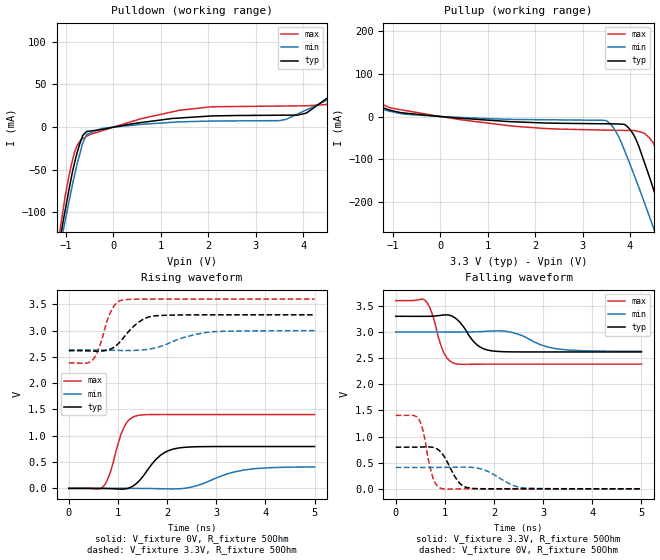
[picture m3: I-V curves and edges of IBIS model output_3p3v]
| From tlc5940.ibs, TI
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|   output_3p3v Model
[Model]   output_3p3v
Model_type   Output
Polarity   Non-Inverting
Vmeas = 1.65
Vref = 1.65
Cref = 15pF
Rref = 50
|   typ   min   max
|   (nom PVT)   (Fast PVT)   (slow PVT)
|Average
C_comp   1.731e-12   1.729e-12   1.773e-12
|ON state : BUFFER OUTPUT TURNED HIGH
|C_comp   1.838e-12   1.835e-12   1.905e-12
|OFF state: BUFFER is in LOW state
|C_comp   1.628e-12   1.621e-12   1.641e-12
| Where nom  PVT is Nominal Process, 3.3V, 65C
|   Fast PVT is Strong Process,  3.6V, -40C
|   Slow PVT is Weak Process,   3V, 125C
[Voltage Range]   3.3   3   3.6
|Ambient Temperature   25   85   -40
|Junction Temperature
[Temperature Range]   65   125   -40
[Pullup Reference]   3.3   3   3.6
[Pulldown Reference]   0   0   0
[Power Clamp Reference]   3.3   3   3.6
[GND Clamp Reference]   0   0   0
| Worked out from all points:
|   slope of the pulldown table from 0 to 0.495 V, typ, clamps not added: 104 ohm
|   slope of the pullup table from 0 to 0.495 V, typ, clamps not added: 107 ohm
|   falling waveform, V_fixture 3.3V, R_fixture 50Ohm: 20-80 % time 327ps typ, 545ps min, 229ps max; typ from 3.3 V to 2.62 V
|   rising waveform, V_fixture 0V, R_fixture 50Ohm: 20-80 % time 430ps typ, 735ps min, 270ps max; typ from 0 V to 0.796 V
|   rising waveform, V_fixture 3.3V, R_fixture 50Ohm: 20-80 % time 417ps typ, 697ps min, 255ps max; typ from 2.62 V to 3.3 V
|   falling waveform, V_fixture 0V, R_fixture 50Ohm: 20-80 % time 284ps typ, 463ps min, 183ps max; typ from 0.796 V to 0 V
[Pulldown]
|   Voltage   I(typ)   I(min)   I(max)
-3.3V     -940.2mA   -857.4mA   -1.084A
-1.139V   -135.7mA   -144.9mA   -125.6mA
-1.092V   -120.7mA   -131mA     -108.3mA
-1.046V   -105.9mA   -117.8mA   -91.31mA
-823.2mV  -42.75mA   -57.22mA   -30.01mA
-564mV    -5.078mA   -8.618mA   -10.77mA
1.398V    10.71mA    6.227mA    19.78mA
3.498V    13.98mA    7.63mA     24.69mA
4.066V    16.44mA    20.12mA    25.02mA
4.49V     33.36mA    31.46mA    26.46mA
4.814V    46.59mA    40.99mA    50.25mA
6.6V      125.7mA    93.65mA    209.8mA
[Pullup]
|   Voltage   I(typ)   I(min)   I(max)
-3.3V     110.7mA    76.62mA    210.2mA
-1.061V   14.71mA    12.28mA    20.6mA
1.538V    -12.39mA   -6.887mA   -22.73mA
3.498V    -17.16mA   -9.56mA    -32.01mA
3.759V    -17.69mA   -47mA      -32.48mA
4.019V    -33.45mA   -117.8mA   -32.94mA
4.188V    -70.87mA   -167.3mA   -35.65mA
4.487V    -168.3mA   -259.4mA   -61.5mA
4.752V    -259.4mA   -344mA     -158mA
4.926V    -322.2mA   -400.7mA   -230.3mA
5.115V    -390.5mA   -463.1mA   -311.7mA
6.6V      -960mA     -972.2mA   -980.3mA
[Ramp]
R_load = 50
|   typ   min   max
dV/dt_r   0.477664/4.29009e-10   0.244378/7.25716e-10   0.842488/2.69271e-10
dV/dt_f   0.409109/3.26691e-10   0.221026/5.38551e-10   0.728975/2.28779e-10
[Falling Waveform]
V_fixture = 3.3V
V_fixture_min = 3V
V_fixture_max = 3.6V
R_fixture = 50Ohm
|   Time   V(typ)   V(min)   V(max)
0s        3.3V       3V         3.6V
610ps     3.3V       3V         3.592V
740ps     3.303V     3V         3.354V
980ps     3.326V     3V         2.603V
1.22ns    3.26V      2.999V     2.393V
1.65ns    2.757V     3.005V     2.384V
1.94ns    2.641V     3.018V     2.385V
2.44ns    2.619V     2.973V     2.385V
3.29ns    2.618V     2.676V     2.385V
5ns       2.618V     2.632V     2.385V
[Rising Waveform]
V_fixture = 0V
V_fixture_min = 0V
V_fixture_max = 0V
R_fixture = 50Ohm
|   Time   V(typ)   V(min)   V(max)
0s        217pV      1.746nV    184.6pV
700ps     -1.346mV   318uV      34.54mV
840ps     -4.411mV   391.2uV    296.3mV
1.11ns    -13.2mV    214.7uV    1.137V
1.35ns    73.79mV    -716.1uV   1.372V
1.85ns    617.5mV    -6.212mV   1.404V
2.14ns    750.6mV    -10.1mV    1.404V
2.52ns    789.2mV    30.04mV    1.404V
3.57ns    796.1mV    350.3mV    1.404V
5ns       796.1mV    407.3mV    1.404V
[Rising Waveform]
V_fixture = 3.3V
V_fixture_min = 3V
V_fixture_max = 3.6V
R_fixture = 50Ohm
|   Time   V(typ)   V(min)   V(max)
0s        2.618V     2.631V     2.385V
490ps     2.61V      2.631V     2.447V
620ps     2.608V     2.63V      2.683V
860ps     2.653V     2.626V     3.371V
970ps     2.72V      2.624V     3.524V
1.09ns    2.838V     2.622V     3.582V
1.42ns    3.159V     2.628V     3.598V
1.73ns    3.278V     2.664V     3.6V
2.8ns     3.3V       2.965V     3.6V
5ns       3.3V       3V         3.6V
[Falling Waveform]
V_fixture = 0V
V_fixture_min = 0V
V_fixture_max = 0V
R_fixture = 50Ohm
|   Time   V(typ)   V(min)   V(max)
0s        796.2mV    408.7mV    1.404V
460ps     797.8mV    408.4mV    1.352V
560ps     800.3mV    408.4mV    1.097V
660ps     802mV      408.6mV    576.2mV
760ps     792.8mV    408.9mV    202.6mV
930ps     690.4mV    409.8mV    5.39mV
1.28ns    129.9mV    413.9mV    -929.1uV
1.47ns    19.69mV    413.8mV    185.1uV
2.62ns    97.18uV    15.78mV    226.7uV
5ns       75.05uV    42.81uV    179.4uV
